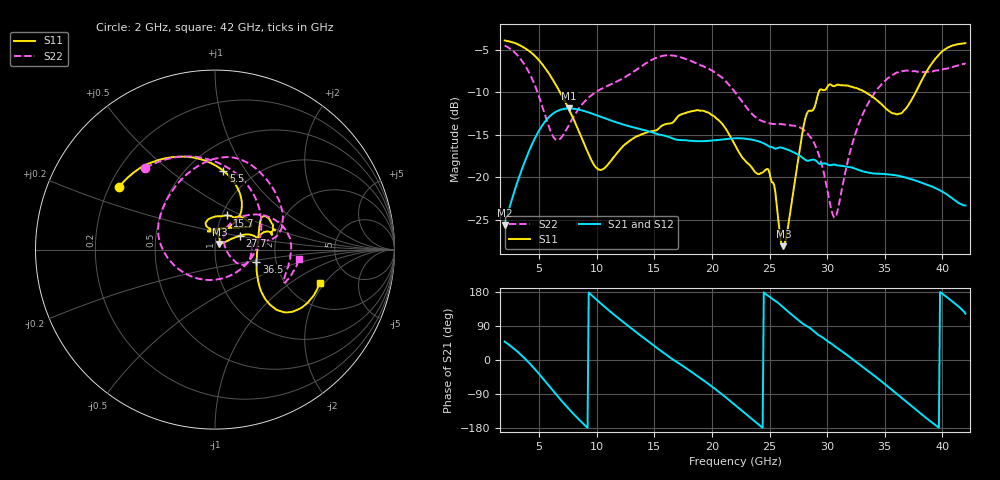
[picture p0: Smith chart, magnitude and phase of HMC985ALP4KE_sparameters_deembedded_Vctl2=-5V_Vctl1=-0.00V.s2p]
!s2p File: Measurements: S11, S21, S12, S22
# GHz S dB R 50.0
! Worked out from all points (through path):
!   401 points, 2 GHz to 42 GHz, reference 50 ohm
!   highest |S21| = -11.89 dB at 7.6 GHz (marker M1); lowest = -25.7 dB at 2 GHz (marker M2)
!   lowest |S11| = -28.1 dB at 26.2 GHz (marker M3), VSWR 1.08, Z = 52.4 + j3.26 ohm
!   |S11| at or under -10 dB: 6.813 GHz to 29.26 GHz (22.45 GHz wide, 124 % of centre); 33.34 GHz to 37.68 GHz (4.346 GHz wide, 12.2 % of centre)
!   |S22| runs from -24.7 to -4.5 dB; largest |S21 - S12| = 0.00023
!   S11 on the Smith chart (normalised r, x): 2 GHz: 0.24, +0.28; 5.5 GHz: 0.73, +0.80; 15.7 GHz: 1.06, +0.42; 27.7 GHz: 1.30, +0.21; 36.5 GHz: 1.58, -0.22; 42 GHz: 3.01, -1.82
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2  -3.89 147.1  -25.65 48.6  -25.66 48.6  -4.48 130.5
3.6  -4.67 120.3  -18.70 8.4  -18.70 8.4  -6.48 84.9
5.5  -7.12 83.9  -13.46 -55.3  -13.47 -55.3  -12.62 2.5
6.5  -9.24 66.6  -12.24 -91.8  -12.25 -91.8  -15.60 -68.6
7.6  -12.05 55.0  -11.89 -129.9  -11.90 -129.9  -13.79 -135.5
8.7  -15.39 55.4  -12.12 -164.5  -12.12 -164.5  -11.46 -170.0
10.4  -19.11 89.8  -12.89 147.8  -12.90 147.8  -9.59 162.7
12.7  -15.87 108.2  -13.95 90.5  -13.95 90.5  -8.02 129.2
15.4  -14.23 75.9  -14.97 27.9  -14.97 28.0  -5.83 87.7
15.7  -13.89 70.6  -15.04 21.3  -15.04 21.3  -5.71 83.8
19.4  -12.25 33.6  -15.73 -56.7  -15.74 -56.6  -7.04 35.7
22  -16.18 51.4  -15.40 -118.6  -15.41 -118.6  -9.98 10.2
24.9  -19.09 104.8  -16.32 168.8  -16.33 168.8  -13.62 13.5
26.2  -28.10 52.2  -16.56 138.3  -16.57 138.3  -13.77 -1.2
27.7  -16.05 29.6  -17.52 100.3  -17.52 100.3  -14.19 -21.6
28.7  -12.15 13.3  -17.92 79.8  -17.92 79.8  -15.53 -30.0
30.7  -9.23 21.3  -18.51 35.6  -18.52 35.6  -24.74 21.7
32.8  -9.65 34.5  -19.16 -12.0  -19.17 -12.0  -13.51 54.6
35.4  -12.21 11.7  -19.66 -73.2  -19.67 -73.2  -8.22 22.3
36.5  -12.41 -16.2  -19.92 -101.0  -19.92 -101.0  -7.48 8.2
39.5  -5.89 -42.8  -21.33 -174.0  -21.34 -173.9  -7.43 -25.0
42  -4.21 -17.7  -23.31 122.2  -23.32 122.1  -6.55 -6.2
